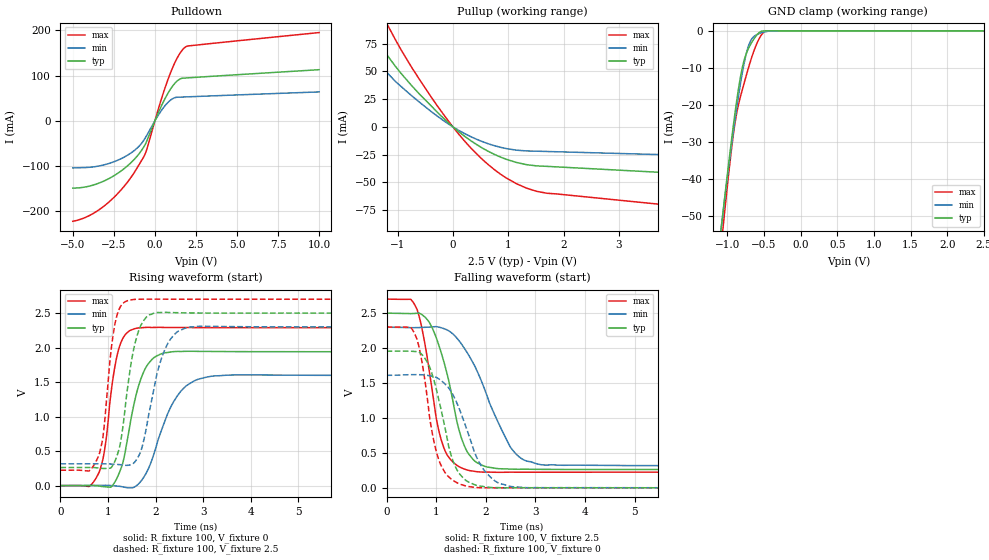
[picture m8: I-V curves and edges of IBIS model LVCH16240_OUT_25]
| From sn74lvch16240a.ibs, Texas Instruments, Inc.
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[Model]   LVCH16240_OUT_25
Model_type  3-state
Enable   Active-Low
Vref =   0
Rref =   500
Cref =   30p
Vmeas =   1.25
| variable   typ   min   max
C_comp   4.81pF   4.38pF   6.01pF
| C_pullup   6.00pF   3.89pF   9.13pF
| C_pulldown   7.53pF   5.42pF   9.58pF
| C_tri-state   4.81pF   4.38pF   6.01pF
[Temperature Range]   40   100   -40
| Ambient temperature   25   85   -40
[Voltage range]   2.5   2.3   2.7
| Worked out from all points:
|   slope of the pulldown table from 0 to 0.375 V, typ, clamps not added: 11.9 ohm
|   slope of the pullup table from 0 to 0.375 V, typ, clamps not added: 26.5 ohm
|   GND clamp passes 1 mA (typ) near -0.59 V on its own axis
|   rising waveform, R_fixture 100, V_fixture 0: 20-80 % time 364ps typ, 543ps min, 261ps max; typ from 0 V to 1.94 V
|   falling waveform, R_fixture 100, V_fixture 2.5: 20-80 % time 463ps typ, 749ps min, 354ps max; typ from 2.5 V to 0.262 V
|   rising waveform, R_fixture 100, V_fixture 2.5: 20-80 % time 281ps typ, 386ps min, 215ps max; typ from 0.262 V to 2.5 V
|   falling waveform, R_fixture 100, V_fixture 0: 20-80 % time 390ps typ, 532ps min, 322ps max; typ from 1.95 V to 0 V
[GND Clamp]
| LVCH16240_OUT_25
|   Voltage   I(typ)   I(min)   I(max)
-5V       -855.7mA   -797.6mA   -953.2mA
-1.09V    -54.36mA   -53.97mA   -59.22mA
-1.06V    -49.06mA   -49.09mA   -53.29mA
-955mV    -31.29mA   -32.66mA   -33.81mA
-900mV    -22.75mA   -24.6mA    -25.4mA
-840mV    -14.58mA   -16.51mA   -19.19mA
-790mV    -9.382mA   -10.63mA   -15.45mA
-730mV    -5.543mA   -5.229mA   -11.2mA
-675mV    -3.361mA   -2.41mA    -7.57mA
-570mV    -549.4uA   -770.8uA   -2.257mA
-490mV    -16.56uA   -280.7uA   -181.4uA
2.5V      9.149pA    38.1nA     -134.7pA
[Pulldown]
| LVCH16240_OUT_25
|   Voltage   I(typ)   I(min)   I(max)
-5V       -148.4mA   -103.9mA   -221.8mA
-4.05V    -144.6mA   -102.7mA   -210.3mA
-3.075V   -132.4mA   -96.92mA   -187.6mA
-2.11V    -112mA     -84.37mA   -154.5mA
-1.27V    -85.53mA   -65.87mA   -114.9mA
-850mV    -67.03mA   -51.33mA   -89.83mA
-540mV    -48.37mA   -34.68mA   -68.09mA
230mV     19.76mA    13.93mA    28.68mA
750mV     58.22mA    39.1mA     86.73mA
1.33V     87.32mA    52.22mA    137mA
1.83V     94.73mA    52.98mA    162.4mA
10V       113.2mA    64.1mA     195.3mA
[Pullup]
| LVCH16240_OUT_25
|   Voltage   I(typ)   I(min)   I(max)
-5V       107mA      39.78mA    366.9mA
-3.895V   252mA      53.48mA    373.6mA
-3.68V    242.4mA    66.07mA    353.2mA
-3.58V    236.9mA    97.7mA     343.4mA
-1.875V   115.8mA    88.65mA    164.7mA
-1.47V    84.95mA    64.9mA     120.5mA
-1.2V     65.32mA    49.39mA    93.48mA
-395mV    18.99mA    13.91mA    27.01mA
320mV     -12.34mA   -8.718mA   -18.78mA
965mV     -29.2mA    -19.52mA   -46.04mA
1.515V    -35.13mA   -21.87mA   -58.07mA
10V       -57.52mA   -33.56mA   -101.4mA
[Ramp]
| LVCH16240_OUT_25
| variable   typ   min   max
dV/dt_r   1.18/3.74E-10   0.98/5.64E-10   1.38/2.68E-10
dV/dt_f   1.34/4.72E-10   1.19/7.67E-10   1.49/3.64E-10
R_load = 100
[Rising Waveform]
| LVCH16240_OUT_25
R_fixture =   100
C_fixture =   0
L_fixture =   0
V_fixture =   0
V_fixture_min = 0
V_fixture_max = 0
|   Time   V(typ)   V(min)   V(max)
0s        166.8uV    4.312uV    373.4uV
805ps     -5.472mV   3.222mV    181.3mV
940ps     -16.61mV   4.57mV     568.3mV
1.115ns   21.03mV    -1.424mV   1.599V
1.34ns    411.7mV    -21.9mV    2.165V
1.575ns   1.267V     -12.27mV   2.276V
1.765ns   1.669V     135.7mV    2.291V
2.53ns    1.943V     1.365V     2.29V
3.52ns    1.942V     1.601V     2.289V
49.99ns   1.941V     1.598V     2.289V
[Falling Waveform]
| LVCH16240_OUT_25
R_fixture =   100
C_fixture =   0
L_fixture =   0
V_fixture =   2.5
V_fixture_min = 2.3
V_fixture_max = 2.7
|   Time   V(typ)   V(min)   V(max)
0s        2.498V     2.298V     2.699V
555ps     2.494V     2.291V     2.631V
855ps     2.373V     2.299V     1.693V
1.025ns   2.096V     2.302V     906.6mV
1.195ns   1.694V     2.265V     501.9mV
1.525ns   676.2mV    2.04V      279.5mV
1.885ns   337.5mV    1.57V      225.8mV
2.515ns   266.5mV    561.4mV    222.8mV
3.19ns    262.9mV    324.7mV    222.5mV
49.99ns   262mV      316.3mV    223.1mV
[Rising Waveform]
| LVCH16240_OUT_25
R_fixture =   100
C_fixture =   0
L_fixture =   0
V_fixture =   2.5
V_fixture_min = 2.3
V_fixture_max = 2.7
|   Time   V(typ)   V(min)   V(max)
0s        262mV      316.2mV    223.1mV
815ps     254.5mV    316.6mV    452.5mV
905ps     249.2mV    316.5mV    764.1mV
1.105ns   299.2mV    311.5mV    2.174V
1.26ns    613.8mV    303.3mV    2.591V
1.58ns    2.092V     357.2mV    2.699V
1.82ns    2.45V      884.2mV    2.702V
2.225ns   2.51V      2.014V     2.701V
2.915ns   2.501V     2.308V     2.7V
49.99ns   2.498V     2.298V     2.699V
[Falling Waveform]
| LVCH16240_OUT_25
R_fixture =   100
C_fixture =   0
L_fixture =   0
V_fixture =   0
V_fixture_min = 0
V_fixture_max = 0
|   Time   V(typ)   V(min)   V(max)
0s        1.953V     1.608V     2.299V
510ps     1.953V     1.619V     2.272V
775ps     1.848V     1.613V     1.517V
925ps     1.608V     1.594V     764.1mV
1.1ns     1.11V      1.532V     316.1mV
1.4ns     280.3mV    1.237V     78.79mV
1.855ns   26.93mV    378.8mV    1.799mV
2.235ns   2.177mV    75.38mV    -1.391mV
2.875ns   335.4uV    -192.7uV   -60.14uV
49.99ns   173uV      63.22uV    351.9uV
